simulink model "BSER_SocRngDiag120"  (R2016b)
settings: Solver=FixedStepDiscrete  StartTime=0.0  StopTime=10.0  FixedStep=0.02  RelTol=1e-3  EnableMultiTasking=on
undefined symbols (not defined in the file or in its folder): bin2dec, BSER_cntSocRngDiag_CW, BSER_iSocRngChCurrAccuThres_C, BSER_iSocRngDisCurrAccuThres_C, BSER_rBattSocRngHiFault_C, BSER_rBattSocRngHiWarn_C, BSER_rBattSocRngLoFault_C, BSER_rBattSocRngLoWarn_C, BSER_tiBattSocRngHiFault_C, BSER_tiBattSocRngHiWarn_C, BSER_tiBattSocRngLoFault_C, BSER_tiBattSocRngLoWarn_C, BSPR_iSocRngChrgCurrHi_C, BSPR_iSocRngDisChCurrLo_C, BSPR_tiSocRngCurrCont_C
libraries: simulink x32

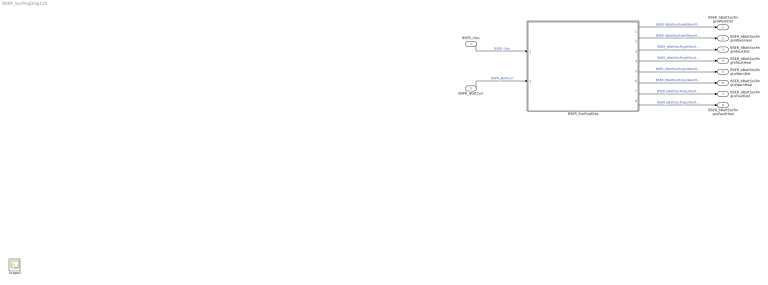
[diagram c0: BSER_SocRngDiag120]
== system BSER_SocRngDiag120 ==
  BSER_rSoc : Inport
  BSPR_iBattCurr : Inport  Port=2
  BSER_SocRngDiag : Subsystem
  BSER_bBattSocRngHiWarnDet : Outport
  BSER_bBattSocRngHiWarnHeal : Outport  Port=2
  BSER_bBattSocRngHiFaultDet : Outport  Port=3
  BSER_bBattSocRngHiFaultHeal : Outport  Port=4
  BSER_bBattSocRngLoWarnDet : Outport  Port=5
  BSER_bBattSocRngLoWarnHeal : Outport  Port=6
  BSER_bBattSocRngLoFaultDet : Outport  Port=7
  BSER_bBattSocRngLoFaultHeal : Outport  Port=8
  Scope2 : Scope
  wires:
  BSER_rSoc/1 -> BSER_SocRngDiag/1(BSER_rSoc)  "BSER_rSoc"
  BSPR_iBattCurr/1 -> BSER_SocRngDiag/2(BSPR_iBattCurr)  "BSPR_iBattCurr"
  BSER_SocRngDiag/1(BSER_bBattSocRngHiWarnDet) -> BSER_bBattSocRngHiWarnDet/1  "BSER_bBattSocRngHiWarnDet"
  BSER_SocRngDiag/2(BSER_bBattSocRngHiWarnHeal) -> BSER_bBattSocRngHiWarnHeal/1  "BSER_bBattSocRngHiWarnHeal"
  BSER_SocRngDiag/3(BSER_bBattSocRngHiFaultDet) -> BSER_bBattSocRngHiFaultDet/1  "BSER_bBattSocRngHiFaultDet"
  BSER_SocRngDiag/4(BSER_bBattSocRngHiFaultHeal) -> BSER_bBattSocRngHiFaultHeal/1  "BSER_bBattSocRngHiFaultHeal"
  BSER_SocRngDiag/5(BSER_bBattSocRngLoWarnDet) -> BSER_bBattSocRngLoWarnDet/1  "BSER_bBattSocRngLoWarnDet"
  BSER_SocRngDiag/6(BSER_bBattSocRngLoWarnHeal) -> BSER_bBattSocRngLoWarnHeal/1  "BSER_bBattSocRngLoWarnHeal"
  BSER_SocRngDiag/7(BSER_bBattSocRngLoFaultDet) -> BSER_bBattSocRngLoFaultDet/1  "BSER_bBattSocRngLoFaultDet"
  BSER_SocRngDiag/8(BSER_bBattSocRngLoFaultHeal) -> BSER_bBattSocRngLoFaultHeal/1  "BSER_bBattSocRngLoFaultHeal"

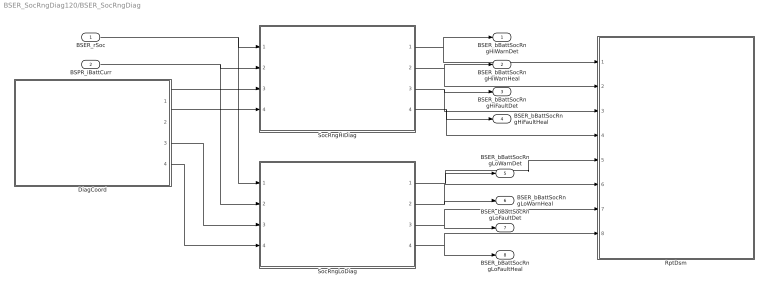
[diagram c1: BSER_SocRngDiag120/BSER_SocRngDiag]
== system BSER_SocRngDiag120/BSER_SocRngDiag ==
  BSER_rSoc : Inport
  BSPR_iBattCurr : Inport  Port=2
  DiagCoord : Subsystem
  RptDsm : Subsystem
  SocRngHiDiag : Subsystem
  SocRngLoDiag : Subsystem
  BSER_bBattSocRngHiWarnDet : Outport
  BSER_bBattSocRngHiWarnHeal : Outport  Port=2
  BSER_bBattSocRngHiFaultDet : Outport  Port=3
  BSER_bBattSocRngHiFaultHeal : Outport  Port=4
  BSER_bBattSocRngLoWarnDet : Outport  Port=5
  BSER_bBattSocRngLoWarnHeal : Outport  Port=6
  BSER_bBattSocRngLoFaultDet : Outport  Port=7
  BSER_bBattSocRngLoFaultHeal : Outport  Port=8
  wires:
  BSER_rSoc/1 -> SocRngHiDiag/1(BSER_rSoc), SocRngLoDiag/1(BSER_rSoc)
  BSPR_iBattCurr/1 -> SocRngHiDiag/2(BSPR_iBattCurr), SocRngLoDiag/2(BSPR_iBattCurr)
  DiagCoord/1(BSPR_bSocRngHiWarnSwt) -> SocRngHiDiag/3(BSPR_bSocRngHiWarnSwt)
  DiagCoord/2(BSPR_bSocRngHiFaultSwt) -> SocRngHiDiag/4(BSPR_bSocRngHiFaultSwt)
  SocRngHiDiag/1(BSER_bBattSocRngHiWarnDet) -> RptDsm/1(BSER_bBattSocRngHiWarnDet), BSER_bBattSocRngHiWarnDet/1
  SocRngHiDiag/2(BSER_bBattSocRngHiWarnHeal) -> RptDsm/2(BSER_bBattSocRngHiWarnHeal), BSER_bBattSocRngHiWarnHeal/1
  DiagCoord/3(BSPR_bSocRngLoWarnSwt) -> SocRngLoDiag/3(BSPR_bSocRngLoWarnSwt)
  DiagCoord/4(BSPR_bSocRngLoFaultSwt) -> SocRngLoDiag/4(BSPR_bSocRngLoFaultSwt)
  SocRngLoDiag/1(BSER_bBattSocRngLoWarnDet) -> RptDsm/5(BSER_bBattSocRngLoWarnDet), BSER_bBattSocRngLoWarnDet/1
  SocRngLoDiag/2(BSER_bBattSocRngLoWarnHeal) -> RptDsm/6(BSER_bBattSocRngLoWarnHeal), BSER_bBattSocRngLoWarnHeal/1
  SocRngHiDiag/3(BSER_bBattSocRngHiFaultDet) -> RptDsm/3(BSER_bBattSocRngHiFaultDet), BSER_bBattSocRngHiFaultDet/1
  SocRngHiDiag/4(BSER_bBattSocRngHiFaultHeal) -> RptDsm/4(BSER_bBattSocRngHiFaultHeal), BSER_bBattSocRngHiFaultHeal/1
  SocRngLoDiag/3(BSER_bBattSocRngLoFaultDet) -> RptDsm/7(BSER_bBattSocRngLoFaultDet), BSER_bBattSocRngLoFaultDet/1
  SocRngLoDiag/4(BSER_bBattSocRngLoFaultHeal) -> BSER_bBattSocRngLoFaultHeal/1, RptDsm/8(BSER_bBattSocRngLoFaultHeal)

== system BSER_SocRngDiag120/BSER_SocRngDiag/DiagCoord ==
  Bitwise Operator : simulink/Logic and Bit Operations/Bitwise Operator  logicop=AND  UseBitMask=on  BitMask=bin2dec('00000001')  BitMaskRealWorld=Stored Integer
  Bitwise Operator1 : simulink/Logic and Bit Operations/Bitwise Operator  logicop=AND  UseBitMask=on  BitMask=bin2dec('00000010')  BitMaskRealWorld=Stored Integer
  Bitwise Operator2 : simulink/Logic and Bit Operations/Bitwise Operator  logicop=AND  UseBitMask=on  BitMask=bin2dec('00000100')  BitMaskRealWorld=Stored Integer
  Bitwise Operator3 : simulink/Logic and Bit Operations/Bitwise Operator  logicop=AND  UseBitMask=on  BitMask=bin2dec('00001000')  BitMaskRealWorld=Stored Integer
  Compare To Constant : simulink/Logic and Bit Operations/Compare To Constant  relop===  const=1  OutDataTypeStr=boolean
  Compare To Constant1 : simulink/Logic and Bit Operations/Compare To Constant  relop===  const=2  OutDataTypeStr=boolean
  Compare To Constant2 : simulink/Logic and Bit Operations/Compare To Constant  relop===  const=4  OutDataTypeStr=boolean
  Compare To Constant3 : simulink/Logic and Bit Operations/Compare To Constant  relop===  const=8  OutDataTypeStr=boolean
  Constant7 : Constant  Value=BSER_cntSocRngDiag_CW
  BSPR_bSocRngHiWarnSwt : Outport
  BSPR_bSocRngHiFaultSwt : Outport  Port=2
  BSPR_bSocRngLoWarnSwt : Outport  Port=3
  BSPR_bSocRngLoFaultSwt : Outport  Port=4
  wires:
  Compare To Constant/1 -> BSPR_bSocRngHiWarnSwt/1  "BSPR_bSocRngHiWarnSwt"
  Compare To Constant1/1 -> BSPR_bSocRngHiFaultSwt/1  "BSPR_bSocRngHiFaultSwt"
  Compare To Constant2/1 -> BSPR_bSocRngLoWarnSwt/1  "BSPR_bSocRngLoWarnSwt"
  Compare To Constant3/1 -> BSPR_bSocRngLoFaultSwt/1  "BSPR_bSocRngLoFaultSwt"
  Constant7/1 -> Bitwise Operator3/1, Bitwise Operator2/1, Bitwise Operator1/1, Bitwise Operator/1
  Bitwise Operator/1 -> Compare To Constant/1
  Bitwise Operator1/1 -> Compare To Constant1/1
  Bitwise Operator2/1 -> Compare To Constant2/1
  Bitwise Operator3/1 -> Compare To Constant3/1

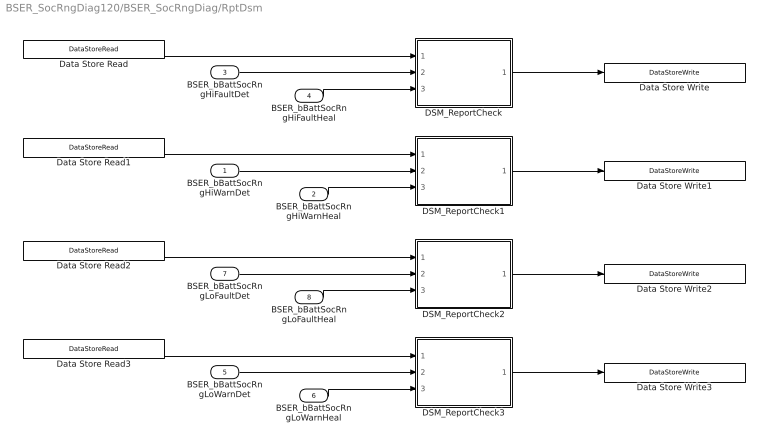
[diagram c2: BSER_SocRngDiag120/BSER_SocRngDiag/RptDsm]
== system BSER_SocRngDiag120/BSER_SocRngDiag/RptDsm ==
  BSER_bBattSocRngHiWarnDet : Inport
  BSER_bBattSocRngHiWarnHeal : Inport  Port=2
  BSER_bBattSocRngHiFaultDet : Inport  Port=3
  BSER_bBattSocRngHiFaultHeal : Inport  Port=4
  BSER_bBattSocRngLoWarnDet : Inport  Port=5
  BSER_bBattSocRngLoWarnHeal : Inport  Port=6
  BSER_bBattSocRngLoFaultDet : Inport  Port=7
  BSER_bBattSocRngLoFaultHeal : Inport  Port=8
  DSM_ReportCheck : Subsystem  TreatAsAtomicUnit=on  RTWFcnName=DSM_ReportCheck  RTWFileName=SrvLib
  DSM_ReportCheck1 : Subsystem  TreatAsAtomicUnit=on  RTWFcnName=DSM_ReportCheck  RTWFileName=SrvLib
  DSM_ReportCheck2 : Subsystem  TreatAsAtomicUnit=on  RTWFcnName=DSM_ReportCheck  RTWFileName=SrvLib
  DSM_ReportCheck3 : Subsystem  TreatAsAtomicUnit=on  RTWFcnName=DSM_ReportCheck  RTWFileName=SrvLib
  Data Store Read : DataStoreRead  DataStoreName=DFC_SocRngHiMax
  Data Store Read1 : DataStoreRead  DataStoreName=DFC_SocRngHiMin
  Data Store Read2 : DataStoreRead  DataStoreName=DFC_SocRngLoMax
  Data Store Read3 : DataStoreRead  DataStoreName=DFC_SocRngLoMin
  Data Store Write : DataStoreWrite  DataStoreName=DFC_SocRngHiMax
  Data Store Write1 : DataStoreWrite  DataStoreName=DFC_SocRngHiMin
  Data Store Write2 : DataStoreWrite  DataStoreName=DFC_SocRngLoMax
  Data Store Write3 : DataStoreWrite  DataStoreName=DFC_SocRngLoMin
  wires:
  BSER_bBattSocRngHiFaultHeal/1 -> DSM_ReportCheck/3(Heal)
  BSER_bBattSocRngHiFaultDet/1 -> DSM_ReportCheck/2(Err)
  BSER_bBattSocRngHiWarnHeal/1 -> DSM_ReportCheck1/3(Heal)
  BSER_bBattSocRngHiWarnDet/1 -> DSM_ReportCheck1/2(Err)
  BSER_bBattSocRngLoWarnDet/1 -> DSM_ReportCheck3/2(Err)
  BSER_bBattSocRngLoWarnHeal/1 -> DSM_ReportCheck3/3(Heal)
  BSER_bBattSocRngLoFaultDet/1 -> DSM_ReportCheck2/2(Err)
  BSER_bBattSocRngLoFaultHeal/1 -> DSM_ReportCheck2/3(Heal)
  Data Store Read/1 -> DSM_ReportCheck/1(Dfc_id_nv)
  Data Store Read1/1 -> DSM_ReportCheck1/1(Dfc_id_nv)
  Data Store Read2/1 -> DSM_ReportCheck2/1(Dfc_id_nv)
  Data Store Read3/1 -> DSM_ReportCheck3/1(Dfc_id_nv)
  DSM_ReportCheck/1(Dfc_id) -> Data Store Write/1
  DSM_ReportCheck1/1(Dfc_id) -> Data Store Write1/1
  DSM_ReportCheck2/1(Dfc_id) -> Data Store Write2/1
  DSM_ReportCheck3/1(Dfc_id) -> Data Store Write3/1

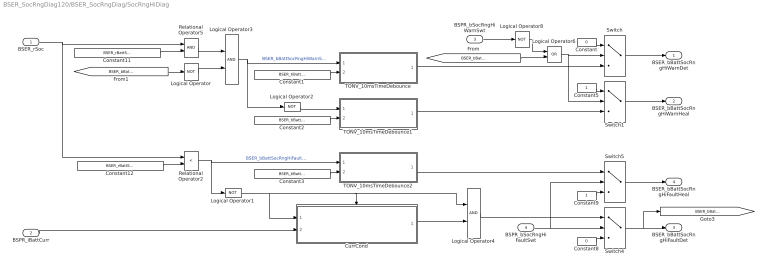
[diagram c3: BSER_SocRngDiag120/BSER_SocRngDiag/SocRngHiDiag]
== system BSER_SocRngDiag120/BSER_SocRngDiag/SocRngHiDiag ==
  BSER_rSoc : Inport
  BSPR_iBattCurr : Inport  Port=2
  BSPR_bSocRngHiWarnSwt : Inport  Port=3
  BSPR_bSocRngHiFaultSwt : Inport  Port=4
  Constant : Constant  Value=0  OutDataTypeStr=boolean
  Constant1 : Constant  Value=BSER_tiBattSocRngHiWarn_C
  Constant11 : Constant  Value=BSER_rBattSocRngHiWarn_C
  Constant12 : Constant  Value=BSER_rBattSocRngHiFault_C
  Constant2 : Constant  Value=BSER_tiBattSocRngHiWarn_C
  Constant3 : Constant  Value=BSER_tiBattSocRngHiFault_C
  Constant5 : Constant  OutDataTypeStr=boolean
  Constant8 : Constant  Value=0  OutDataTypeStr=boolean
  Constant9 : Constant  OutDataTypeStr=boolean
  CurrCond : Subsystem
  Logical Operator{,1..2,8} (4 alike) : Logic  Operator=NOT  AllPortsSameDT=off  OutDataTypeStr=boolean
  Logical Operator3 : Logic  AllPortsSameDT=off  OutDataTypeStr=boolean
  Logical Operator4 : Logic  AllPortsSameDT=off  OutDataTypeStr=boolean
  Logical Operator6 : Logic  Operator=OR  AllPortsSameDT=off  OutDataTypeStr=boolean
  Relational Operator2 : RelationalOperator  Operator=<  OutDataTypeStr=boolean  RndMeth=Simplest
  Relational Operator5 : RelationalOperator  OutDataTypeStr=boolean  RndMeth=Simplest
  Switch{,1,4..5} (4 alike) : Switch  Criteria=u2 > Threshold
  TONV_10msTimeDebounce : Subsystem  TreatAsAtomicUnit=on  RTWFcnName=TONV_10msTimeDebounce  RTWFileName=SrvLib
  TONV_10msTimeDebounce1 : Subsystem  TreatAsAtomicUnit=on  RTWFcnName=TONV_10msTimeDebounce  RTWFileName=SrvLib
  TONV_10msTimeDebounce2 : Subsystem  TreatAsAtomicUnit=on  RTWFcnName=TONV_10msTimeDebounce  RTWFileName=SrvLib
  BSER_bBattSocRngHiWarnDet : Outport
  BSER_bBattSocRngHiWarnHeal : Outport  Port=2
  BSER_bBattSocRngHiFaultDet : Outport  Port=3
  BSER_bBattSocRngHiFaultHeal : Outport  Port=4
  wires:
  BSER_rSoc/1 -> Relational Operator2/1, Relational Operator5/1
  Constant11/1 -> Relational Operator5/2
  Constant1/1 -> TONV_10msTimeDebounce/2(T)
  Constant12/1 -> Relational Operator2/2
  Relational Operator5/1 -> Logical Operator3/1
  Logical Operator3/1 -> TONV_10msTimeDebounce/1(u), Logical Operator2/1  "BSER_bBattSocRngHiWarnStt"
  Constant2/1 -> TONV_10msTimeDebounce1/2(T)
  Logical Operator2/1 -> TONV_10msTimeDebounce1/1(u)
  Switch/1 -> BSER_bBattSocRngHiWarnDet/1
  Switch1/1 -> BSER_bBattSocRngHiWarnHeal/1
  TONV_10msTimeDebounce1/1(y) -> Switch1/3
  Logical Operator4/1 -> Switch4/1
  Constant8/1 -> Switch4/3
  TONV_10msTimeDebounce2/1(y) -> Switch5/1
  Constant9/1 -> Switch5/3
  Switch5/1 -> BSER_bBattSocRngHiFaultHeal/1
  Switch4/1 -> [BSER_bBattSocRngHiFaultDet], BSER_bBattSocRngHiFaultDet/1
  Logical Operator6/1 -> Switch1/2, Switch/2
  [BSER_bBattSocRngHiFaultDet] -> Logical Operator6/2
  Logical Operator8/1 -> Logical Operator6/1
  Constant/1 -> Switch/1
  TONV_10msTimeDebounce/1(y) -> Switch/3
  Constant5/1 -> Switch1/1
  Logical Operator/1 -> Logical Operator3/2
  BSPR_bSocRngHiWarnSwt/1 -> Logical Operator8/1
  [BSER_bBattSocRngHiFaultDet] -> Logical Operator/1
  BSPR_bSocRngHiFaultSwt/1 -> Switch5/2, Switch4/2
  Relational Operator2/1 -> TONV_10msTimeDebounce2/1(u), Logical Operator1/1  "BSER_bBattSocRngHiFaultStt"
  Constant3/1 -> TONV_10msTimeDebounce2/2(T)
  BSPR_iBattCurr/1 -> CurrCond/2(BSPR_iBattCurr)
  CurrCond/1(BSPR_bSocRngChrgCurrCond) -> Logical Operator4/2
  Logical Operator1/1 -> CurrCond/1(BSER_bBattSocRngHiFaultStt), CurrCond/Enable, Logical Operator4/1

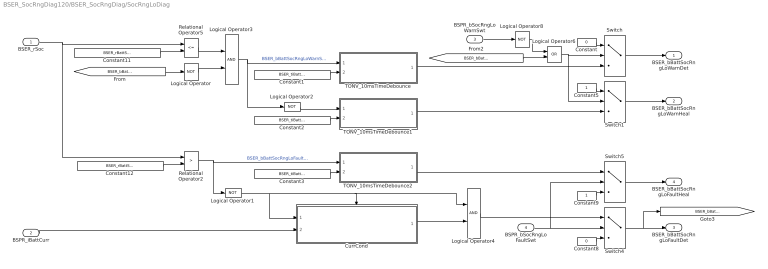
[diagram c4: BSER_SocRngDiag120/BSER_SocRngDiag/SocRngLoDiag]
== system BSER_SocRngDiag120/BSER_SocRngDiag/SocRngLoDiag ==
  BSER_rSoc : Inport
  BSPR_iBattCurr : Inport  Port=2
  BSPR_bSocRngLoWarnSwt : Inport  Port=3
  BSPR_bSocRngLoFaultSwt : Inport  Port=4
  Constant : Constant  Value=0  OutDataTypeStr=boolean
  Constant1 : Constant  Value=BSER_tiBattSocRngLoWarn_C
  Constant11 : Constant  Value=BSER_rBattSocRngLoWarn_C
  Constant12 : Constant  Value=BSER_rBattSocRngLoFault_C
  Constant2 : Constant  Value=BSER_tiBattSocRngLoWarn_C
  Constant3 : Constant  Value=BSER_tiBattSocRngLoFault_C
  Constant5 : Constant  OutDataTypeStr=boolean
  Constant8 : Constant  Value=0  OutDataTypeStr=boolean
  Constant9 : Constant  OutDataTypeStr=boolean
  CurrCond : Subsystem
  Logical Operator{,1..2,8} (4 alike) : Logic  Operator=NOT  AllPortsSameDT=off  OutDataTypeStr=boolean
  Logical Operator3 : Logic  AllPortsSameDT=off  OutDataTypeStr=boolean
  Logical Operator4 : Logic  AllPortsSameDT=off  OutDataTypeStr=boolean
  Logical Operator6 : Logic  Operator=OR  AllPortsSameDT=off  OutDataTypeStr=boolean
  Relational Operator2 : RelationalOperator  Operator=>  OutDataTypeStr=boolean  RndMeth=Simplest
  Relational Operator5 : RelationalOperator  Operator=<=  OutDataTypeStr=boolean  RndMeth=Simplest
  Switch{,1,4..5} (4 alike) : Switch  Criteria=u2 > Threshold
  TONV_10msTimeDebounce : Subsystem  TreatAsAtomicUnit=on  RTWFcnName=TONV_10msTimeDebounce  RTWFileName=SrvLib
  TONV_10msTimeDebounce1 : Subsystem  TreatAsAtomicUnit=on  RTWFcnName=TONV_10msTimeDebounce  RTWFileName=SrvLib
  TONV_10msTimeDebounce2 : Subsystem  TreatAsAtomicUnit=on  RTWFcnName=TONV_10msTimeDebounce  RTWFileName=SrvLib
  BSER_bBattSocRngLoWarnDet : Outport
  BSER_bBattSocRngLoWarnHeal : Outport  Port=2
  BSER_bBattSocRngLoFaultDet : Outport  Port=3
  BSER_bBattSocRngLoFaultHeal : Outport  Port=4
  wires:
  Logical Operator1/1 -> CurrCond/1(BSER_bBattSocRngLo), CurrCond/Enable, Logical Operator4/1
  CurrCond/1(BSPR_bSocRngDisChCurrCond) -> Logical Operator4/2
  BSPR_iBattCurr/1 -> CurrCond/2(BSPR_iBattCurr)
  Constant3/1 -> TONV_10msTimeDebounce2/2(T)
  Relational Operator2/1 -> TONV_10msTimeDebounce2/1(u), Logical Operator1/1  "BSER_bBattSocRngLoFaultStt"
  BSPR_bSocRngLoFaultSwt/1 -> Switch4/2, Switch5/2
  [BSER_bBattSocRngLoFaultDet] -> Logical Operator/1
  BSPR_bSocRngLoWarnSwt/1 -> Logical Operator8/1
  Logical Operator/1 -> Logical Operator3/2
  Constant5/1 -> Switch1/1
  TONV_10msTimeDebounce/1(y) -> Switch/3
  Constant/1 -> Switch/1
  Logical Operator8/1 -> Logical Operator6/1
  [BSER_bBattSocRngLoFaultDet] -> Logical Operator6/2
  Logical Operator6/1 -> Switch/2, Switch1/2
  Switch4/1 -> BSER_bBattSocRngLoFaultDet/1, [BSER_bBattSocRngLoFaultDet]
  Switch5/1 -> BSER_bBattSocRngLoFaultHeal/1
  Constant9/1 -> Switch5/3
  TONV_10msTimeDebounce2/1(y) -> Switch5/1
  Constant8/1 -> Switch4/3
  Logical Operator4/1 -> Switch4/1
  TONV_10msTimeDebounce1/1(y) -> Switch1/3
  Switch1/1 -> BSER_bBattSocRngLoWarnHeal/1
  Switch/1 -> BSER_bBattSocRngLoWarnDet/1
  Logical Operator2/1 -> TONV_10msTimeDebounce1/1(u)
  Constant2/1 -> TONV_10msTimeDebounce1/2(T)
  Logical Operator3/1 -> TONV_10msTimeDebounce/1(u), Logical Operator2/1  "BSER_bBattSocRngLoWarnStt"
  Relational Operator5/1 -> Logical Operator3/1
  Constant12/1 -> Relational Operator2/2
  Constant1/1 -> TONV_10msTimeDebounce/2(T)
  Constant11/1 -> Relational Operator5/2
  BSER_rSoc/1 -> Relational Operator5/1, Relational Operator2/1

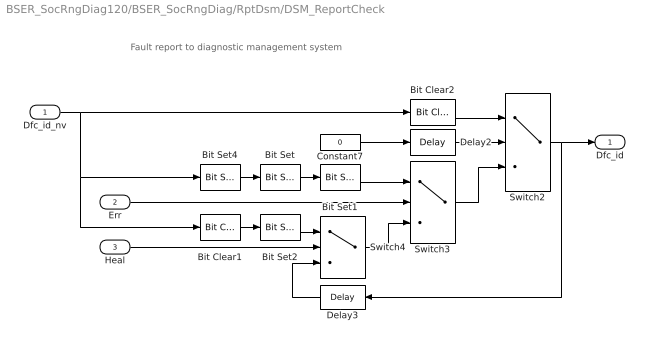
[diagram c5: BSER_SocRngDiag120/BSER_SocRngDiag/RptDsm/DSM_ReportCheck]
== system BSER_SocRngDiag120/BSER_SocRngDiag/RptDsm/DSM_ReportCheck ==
  note: Fault report to diagnostic management system
  Dfc_id_nv : Inport  OutDataTypeStr=uint8
  Err : Inport  Port=2
  Heal : Inport  Port=3
  Bit Clear1 : simulink/Logic and Bit Operations/Bit Clear  iBit=4
  Bit Clear2 : simulink/Logic and Bit Operations/Bit Clear  iBit=3
  Bit Set : simulink/Logic and Bit Operations/Bit Set  iBit=4
  Bit Set1 : simulink/Logic and Bit Operations/Bit Set  iBit=3
  Bit Set2 : simulink/Logic and Bit Operations/Bit Set  iBit=3
  Bit Set4 : simulink/Logic and Bit Operations/Bit Set  iBit=7
  Constant7 : Constant  Value=0  OutDataTypeStr=boolean
  Delay2 : Delay  DelayLength=1  InitialCondition=1
  Delay3 : Delay  DelayLength=1  InitialCondition=0
  Switch2 : Switch  Criteria=u2 ~= 0
  Switch3 : Switch  Criteria=u2 ~= 0
  Switch4 : Switch  Criteria=u2 ~= 0
  Dfc_id : Outport  OutDataTypeStr=uint8
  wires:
  Dfc_id_nv/1 -> Bit Clear2/1, Bit Set4/1, Bit Clear1/1
  Bit Set4/1 -> Bit Set/1
  Constant7/1 -> Delay2/1
  Delay2/1 -> Switch2/2
  Switch3/1 -> Switch2/3
  Bit Clear2/1 -> Switch2/1
  Switch2/1 -> Delay3/1, Dfc_id/1
  Bit Set1/1 -> Switch3/1
  Bit Set/1 -> Bit Set1/1
  Switch4/1 -> Switch3/3
  Err/1 -> Switch3/2
  Bit Set2/1 -> Switch4/1
  Bit Clear1/1 -> Bit Set2/1
  Delay3/1 -> Switch4/3
  Heal/1 -> Switch4/2

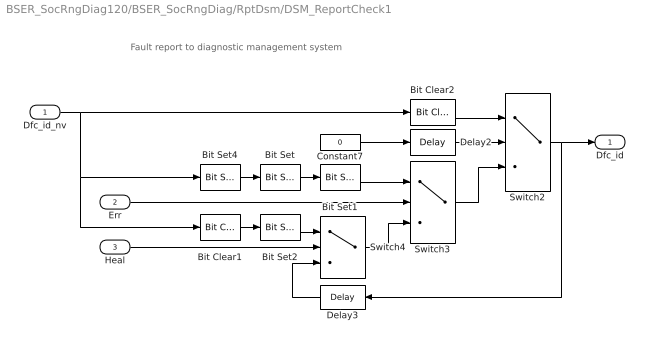
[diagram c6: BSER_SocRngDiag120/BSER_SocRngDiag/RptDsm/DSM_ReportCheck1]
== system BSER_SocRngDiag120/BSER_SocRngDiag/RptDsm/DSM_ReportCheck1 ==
  note: Fault report to diagnostic management system
  Dfc_id_nv : Inport  OutDataTypeStr=uint8
  Err : Inport  Port=2
  Heal : Inport  Port=3
  Bit Clear1 : simulink/Logic and Bit Operations/Bit Clear  iBit=4
  Bit Clear2 : simulink/Logic and Bit Operations/Bit Clear  iBit=3
  Bit Set : simulink/Logic and Bit Operations/Bit Set  iBit=4
  Bit Set1 : simulink/Logic and Bit Operations/Bit Set  iBit=3
  Bit Set2 : simulink/Logic and Bit Operations/Bit Set  iBit=3
  Bit Set4 : simulink/Logic and Bit Operations/Bit Set  iBit=7
  Constant7 : Constant  Value=0  OutDataTypeStr=boolean
  Delay2 : Delay  DelayLength=1  InitialCondition=1
  Delay3 : Delay  DelayLength=1  InitialCondition=0
  Switch2 : Switch  Criteria=u2 ~= 0
  Switch3 : Switch  Criteria=u2 ~= 0
  Switch4 : Switch  Criteria=u2 ~= 0
  Dfc_id : Outport  OutDataTypeStr=uint8
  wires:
  Heal/1 -> Switch4/2
  Delay3/1 -> Switch4/3
  Bit Clear1/1 -> Bit Set2/1
  Bit Set2/1 -> Switch4/1
  Err/1 -> Switch3/2
  Switch4/1 -> Switch3/3
  Bit Set/1 -> Bit Set1/1
  Bit Set1/1 -> Switch3/1
  Switch2/1 -> Dfc_id/1, Delay3/1
  Bit Clear2/1 -> Switch2/1
  Switch3/1 -> Switch2/3
  Delay2/1 -> Switch2/2
  Constant7/1 -> Delay2/1
  Bit Set4/1 -> Bit Set/1
  Dfc_id_nv/1 -> Bit Clear1/1, Bit Set4/1, Bit Clear2/1

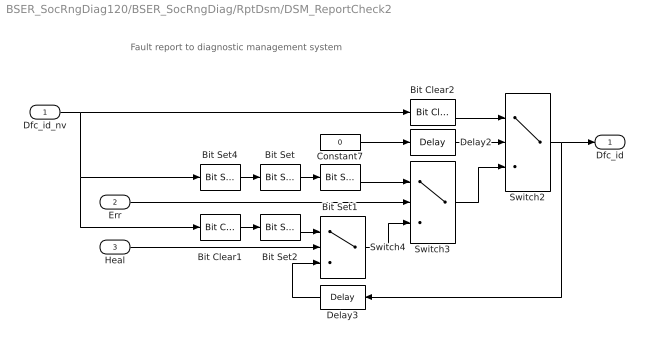
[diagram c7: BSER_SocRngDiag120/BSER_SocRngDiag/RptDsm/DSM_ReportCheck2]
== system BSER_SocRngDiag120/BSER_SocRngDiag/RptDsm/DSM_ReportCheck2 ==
  note: Fault report to diagnostic management system
  Dfc_id_nv : Inport  OutDataTypeStr=uint8
  Err : Inport  Port=2
  Heal : Inport  Port=3
  Bit Clear1 : simulink/Logic and Bit Operations/Bit Clear  iBit=4
  Bit Clear2 : simulink/Logic and Bit Operations/Bit Clear  iBit=3
  Bit Set : simulink/Logic and Bit Operations/Bit Set  iBit=4
  Bit Set1 : simulink/Logic and Bit Operations/Bit Set  iBit=3
  Bit Set2 : simulink/Logic and Bit Operations/Bit Set  iBit=3
  Bit Set4 : simulink/Logic and Bit Operations/Bit Set  iBit=7
  Constant7 : Constant  Value=0  OutDataTypeStr=boolean
  Delay2 : Delay  DelayLength=1  InitialCondition=1
  Delay3 : Delay  DelayLength=1  InitialCondition=0
  Switch2 : Switch  Criteria=u2 ~= 0
  Switch3 : Switch  Criteria=u2 ~= 0
  Switch4 : Switch  Criteria=u2 ~= 0
  Dfc_id : Outport  OutDataTypeStr=uint8
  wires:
  Dfc_id_nv/1 -> Bit Clear2/1, Bit Set4/1, Bit Clear1/1
  Bit Set4/1 -> Bit Set/1
  Constant7/1 -> Delay2/1
  Delay2/1 -> Switch2/2
  Switch3/1 -> Switch2/3
  Bit Clear2/1 -> Switch2/1
  Switch2/1 -> Delay3/1, Dfc_id/1
  Bit Set1/1 -> Switch3/1
  Bit Set/1 -> Bit Set1/1
  Switch4/1 -> Switch3/3
  Err/1 -> Switch3/2
  Bit Set2/1 -> Switch4/1
  Bit Clear1/1 -> Bit Set2/1
  Delay3/1 -> Switch4/3
  Heal/1 -> Switch4/2

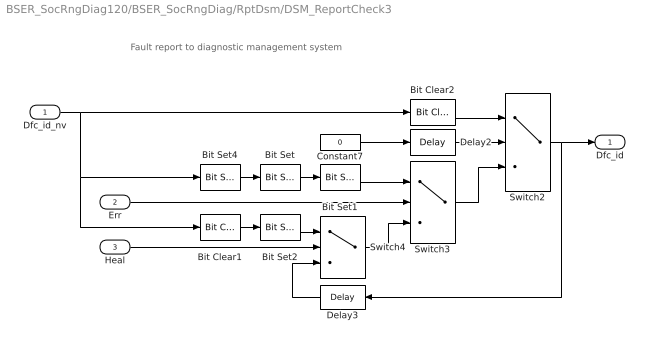
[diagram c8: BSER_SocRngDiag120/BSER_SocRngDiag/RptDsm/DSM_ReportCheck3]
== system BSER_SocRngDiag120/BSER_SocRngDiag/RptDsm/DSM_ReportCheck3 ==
  note: Fault report to diagnostic management system
  Dfc_id_nv : Inport  OutDataTypeStr=uint8
  Err : Inport  Port=2
  Heal : Inport  Port=3
  Bit Clear1 : simulink/Logic and Bit Operations/Bit Clear  iBit=4
  Bit Clear2 : simulink/Logic and Bit Operations/Bit Clear  iBit=3
  Bit Set : simulink/Logic and Bit Operations/Bit Set  iBit=4
  Bit Set1 : simulink/Logic and Bit Operations/Bit Set  iBit=3
  Bit Set2 : simulink/Logic and Bit Operations/Bit Set  iBit=3
  Bit Set4 : simulink/Logic and Bit Operations/Bit Set  iBit=7
  Constant7 : Constant  Value=0  OutDataTypeStr=boolean
  Delay2 : Delay  DelayLength=1  InitialCondition=1
  Delay3 : Delay  DelayLength=1  InitialCondition=0
  Switch2 : Switch  Criteria=u2 ~= 0
  Switch3 : Switch  Criteria=u2 ~= 0
  Switch4 : Switch  Criteria=u2 ~= 0
  Dfc_id : Outport  OutDataTypeStr=uint8
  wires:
  Heal/1 -> Switch4/2
  Delay3/1 -> Switch4/3
  Bit Clear1/1 -> Bit Set2/1
  Bit Set2/1 -> Switch4/1
  Err/1 -> Switch3/2
  Switch4/1 -> Switch3/3
  Bit Set/1 -> Bit Set1/1
  Bit Set1/1 -> Switch3/1
  Switch2/1 -> Dfc_id/1, Delay3/1
  Bit Clear2/1 -> Switch2/1
  Switch3/1 -> Switch2/3
  Delay2/1 -> Switch2/2
  Constant7/1 -> Delay2/1
  Bit Set4/1 -> Bit Set/1
  Dfc_id_nv/1 -> Bit Clear1/1, Bit Set4/1, Bit Clear2/1

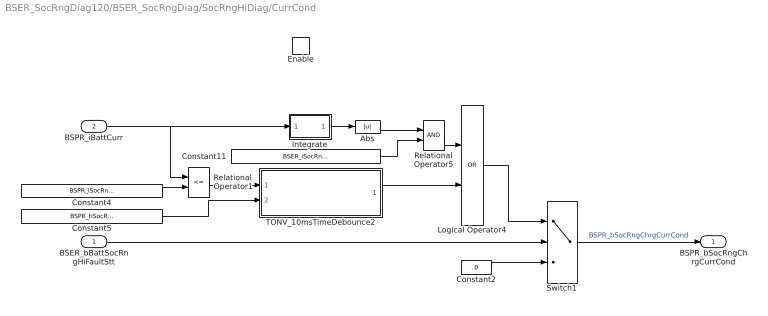
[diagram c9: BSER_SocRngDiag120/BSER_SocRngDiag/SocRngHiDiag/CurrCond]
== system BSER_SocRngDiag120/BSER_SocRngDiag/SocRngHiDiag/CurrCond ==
  BSER_bBattSocRngHiFaultStt : Inport
  BSPR_iBattCurr : Inport  Port=2
  Enable : EnablePort  StatesWhenEnabling=reset
  Abs : Abs
  Constant11 : Constant  Value=BSER_iSocRngChCurrAccuThres_C
  Constant2 : Constant  Value=0  OutDataTypeStr=boolean
  Constant4 : Constant  Value=BSPR_iSocRngChrgCurrHi_C
  Constant5 : Constant  Value=BSPR_tiSocRngCurrCont_C
  Integrate : Subsystem
  Logical Operator4 : Logic  Operator=OR  AllPortsSameDT=off  OutDataTypeStr=boolean
  Relational Operator1 : RelationalOperator  Operator=<=  OutDataTypeStr=boolean  RndMeth=Simplest
  Relational Operator5 : RelationalOperator  OutDataTypeStr=boolean  RndMeth=Simplest
  Switch1 : Switch  Criteria=u2 > Threshold
  TONV_10msTimeDebounce2 : Subsystem  TreatAsAtomicUnit=on  RTWFcnName=TONV_10msTimeDebounce  RTWFileName=SrvLib
  BSPR_bSocRngChrgCurrCond : Outport  InitialOutput=[0]
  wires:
  Integrate/1(Out) -> Abs/1
  Constant11/1 -> Relational Operator5/2
  Constant5/1 -> TONV_10msTimeDebounce2/2(T)
  Constant4/1 -> Relational Operator1/2
  Relational Operator1/1 -> TONV_10msTimeDebounce2/1(u)
  BSER_bBattSocRngHiFaultStt/1 -> Switch1/2
  Constant2/1 -> Switch1/3
  Switch1/1 -> BSPR_bSocRngChrgCurrCond/1  "BSPR_bSocRngChrgCurrCond"
  Logical Operator4/1 -> Switch1/1
  TONV_10msTimeDebounce2/1(y) -> Logical Operator4/2
  Relational Operator5/1 -> Logical Operator4/1
  BSPR_iBattCurr/1 -> Integrate/1(In), Relational Operator1/1
  Abs/1 -> Relational Operator5/1

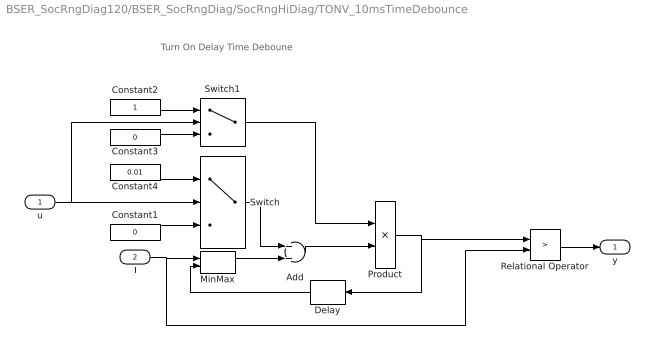
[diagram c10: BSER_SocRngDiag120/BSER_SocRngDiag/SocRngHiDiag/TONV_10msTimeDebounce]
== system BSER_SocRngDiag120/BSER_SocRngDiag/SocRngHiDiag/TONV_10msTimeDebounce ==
  note: Turn On Delay Time Deboune
  u : Inport
  T : Inport  Port=2
  Add : Sum
  Constant1 : Constant  Value=0  OutDataTypeStr=single
  Constant2 : Constant  OutDataTypeStr=uint8
  Constant3 : Constant  Value=0  OutDataTypeStr=uint8
  Constant4 : Constant  Value=0.01  OutDataTypeStr=single
  Delay : Delay  DelayLength=1  InitialCondition=0
  MinMax : MinMax  Inputs=2
  Product : Product  OutMin=[0]  OutMax=[65535]  OutDataTypeStr=single
  Relational Operator : RelationalOperator  Operator=>  OutDataTypeStr=boolean  RndMeth=Simplest
  Switch : Switch  Criteria=u2 ~= 0
  Switch1 : Switch  Criteria=u2 ~= 0
  y : Outport
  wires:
  MinMax/1 -> Add/2
  T/1 -> Relational Operator/2, MinMax/1
  Relational Operator/1 -> y/1
  Delay/1 -> MinMax/2
  Switch/1 -> Add/1
  Product/1 -> Delay/1, Relational Operator/1
  Add/1 -> Product/2
  Constant1/1 -> Switch/3
  Constant4/1 -> Switch/1
  u/1 -> Switch/2, Switch1/2
  Constant2/1 -> Switch1/1
  Constant3/1 -> Switch1/3
  Switch1/1 -> Product/1

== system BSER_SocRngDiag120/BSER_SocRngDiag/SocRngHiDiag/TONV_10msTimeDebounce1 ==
  note: Turn On Delay Time Deboune
  u : Inport
  T : Inport  Port=2
  Add : Sum
  Constant1 : Constant  Value=0  OutDataTypeStr=single
  Constant2 : Constant  OutDataTypeStr=uint8
  Constant3 : Constant  Value=0  OutDataTypeStr=uint8
  Constant4 : Constant  Value=0.01  OutDataTypeStr=single
  Delay : Delay  DelayLength=1  InitialCondition=0
  MinMax : MinMax  Inputs=2
  Product : Product  OutMin=[0]  OutMax=[65535]  OutDataTypeStr=single
  Relational Operator : RelationalOperator  Operator=>  OutDataTypeStr=boolean  RndMeth=Simplest
  Switch : Switch  Criteria=u2 ~= 0
  Switch1 : Switch  Criteria=u2 ~= 0
  y : Outport
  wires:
  Switch1/1 -> Product/1
  Constant3/1 -> Switch1/3
  Constant2/1 -> Switch1/1
  u/1 -> Switch1/2, Switch/2
  Constant4/1 -> Switch/1
  Constant1/1 -> Switch/3
  Add/1 -> Product/2
  Product/1 -> Relational Operator/1, Delay/1
  Switch/1 -> Add/1
  Delay/1 -> MinMax/2
  Relational Operator/1 -> y/1
  T/1 -> MinMax/1, Relational Operator/2
  MinMax/1 -> Add/2

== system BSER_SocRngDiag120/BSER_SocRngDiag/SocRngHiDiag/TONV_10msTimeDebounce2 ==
  note: Turn On Delay Time Deboune
  u : Inport
  T : Inport  Port=2
  Add : Sum
  Constant1 : Constant  Value=0  OutDataTypeStr=single
  Constant2 : Constant  OutDataTypeStr=uint8
  Constant3 : Constant  Value=0  OutDataTypeStr=uint8
  Constant4 : Constant  Value=0.01  OutDataTypeStr=single
  Delay : Delay  DelayLength=1  InitialCondition=0
  MinMax : MinMax  Inputs=2
  Product : Product  OutMin=[0]  OutMax=[65535]  OutDataTypeStr=single
  Relational Operator : RelationalOperator  Operator=>  OutDataTypeStr=boolean  RndMeth=Simplest
  Switch : Switch  Criteria=u2 ~= 0
  Switch1 : Switch  Criteria=u2 ~= 0
  y : Outport
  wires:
  MinMax/1 -> Add/2
  T/1 -> Relational Operator/2, MinMax/1
  Relational Operator/1 -> y/1
  Delay/1 -> MinMax/2
  Switch/1 -> Add/1
  Product/1 -> Delay/1, Relational Operator/1
  Add/1 -> Product/2
  Constant1/1 -> Switch/3
  Constant4/1 -> Switch/1
  u/1 -> Switch/2, Switch1/2
  Constant2/1 -> Switch1/1
  Constant3/1 -> Switch1/3
  Switch1/1 -> Product/1

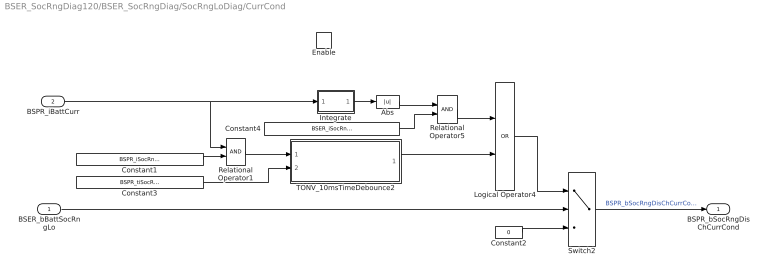
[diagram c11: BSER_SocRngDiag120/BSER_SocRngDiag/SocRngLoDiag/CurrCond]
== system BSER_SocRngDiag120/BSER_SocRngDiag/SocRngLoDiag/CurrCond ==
  BSER_bBattSocRngLo : Inport
  BSPR_iBattCurr : Inport  Port=2
  Enable : EnablePort  StatesWhenEnabling=reset
  Abs : Abs
  Constant1 : Constant  Value=BSPR_iSocRngDisChCurrLo_C
  Constant2 : Constant  Value=0  OutDataTypeStr=boolean
  Constant3 : Constant  Value=BSPR_tiSocRngCurrCont_C
  Constant4 : Constant  Value=BSER_iSocRngDisCurrAccuThres_C
  Integrate : Subsystem
  Logical Operator4 : Logic  Operator=OR  AllPortsSameDT=off  OutDataTypeStr=boolean
  Relational Operator1 : RelationalOperator  OutDataTypeStr=boolean  RndMeth=Simplest
  Relational Operator5 : RelationalOperator  OutDataTypeStr=boolean  RndMeth=Simplest
  Switch2 : Switch  Criteria=u2 > Threshold
  TONV_10msTimeDebounce2 : Subsystem  TreatAsAtomicUnit=on  RTWFcnName=TONV_10msTimeDebounce  RTWFileName=SrvLib
  BSPR_bSocRngDisChCurrCond : Outport  InitialOutput=[0]
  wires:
  Relational Operator5/1 -> Logical Operator4/1
  TONV_10msTimeDebounce2/1(y) -> Logical Operator4/2
  Logical Operator4/1 -> Switch2/1
  Switch2/1 -> BSPR_bSocRngDisChCurrCond/1  "BSPR_bSocRngDisChCurrCond"
  Constant2/1 -> Switch2/3
  BSER_bBattSocRngLo/1 -> Switch2/2
  Relational Operator1/1 -> TONV_10msTimeDebounce2/1(u)
  Constant1/1 -> Relational Operator1/2
  Constant3/1 -> TONV_10msTimeDebounce2/2(T)
  Constant4/1 -> Relational Operator5/2
  Integrate/1(Out) -> Abs/1
  BSPR_iBattCurr/1 -> Integrate/1(In), Relational Operator1/1
  Abs/1 -> Relational Operator5/1

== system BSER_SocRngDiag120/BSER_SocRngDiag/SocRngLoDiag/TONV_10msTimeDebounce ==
  note: Turn On Delay Time Deboune
  u : Inport
  T : Inport  Port=2
  Add : Sum
  Constant1 : Constant  Value=0  OutDataTypeStr=single
  Constant2 : Constant  OutDataTypeStr=uint8
  Constant3 : Constant  Value=0  OutDataTypeStr=uint8
  Constant4 : Constant  Value=0.01  OutDataTypeStr=single
  Delay : Delay  DelayLength=1  InitialCondition=0
  MinMax : MinMax  Inputs=2
  Product : Product  OutMin=[0]  OutMax=[65535]  OutDataTypeStr=single
  Relational Operator : RelationalOperator  Operator=>  OutDataTypeStr=boolean  RndMeth=Simplest
  Switch : Switch  Criteria=u2 ~= 0
  Switch1 : Switch  Criteria=u2 ~= 0
  y : Outport
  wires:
  MinMax/1 -> Add/2
  T/1 -> Relational Operator/2, MinMax/1
  Relational Operator/1 -> y/1
  Delay/1 -> MinMax/2
  Switch/1 -> Add/1
  Product/1 -> Delay/1, Relational Operator/1
  Add/1 -> Product/2
  Constant1/1 -> Switch/3
  Constant4/1 -> Switch/1
  u/1 -> Switch/2, Switch1/2
  Constant2/1 -> Switch1/1
  Constant3/1 -> Switch1/3
  Switch1/1 -> Product/1

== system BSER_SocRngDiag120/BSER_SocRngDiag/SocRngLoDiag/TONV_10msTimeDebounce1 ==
  note: Turn On Delay Time Deboune
  u : Inport
  T : Inport  Port=2
  Add : Sum
  Constant1 : Constant  Value=0  OutDataTypeStr=single
  Constant2 : Constant  OutDataTypeStr=uint8
  Constant3 : Constant  Value=0  OutDataTypeStr=uint8
  Constant4 : Constant  Value=0.01  OutDataTypeStr=single
  Delay : Delay  DelayLength=1  InitialCondition=0
  MinMax : MinMax  Inputs=2
  Product : Product  OutMin=[0]  OutMax=[65535]  OutDataTypeStr=single
  Relational Operator : RelationalOperator  Operator=>  OutDataTypeStr=boolean  RndMeth=Simplest
  Switch : Switch  Criteria=u2 ~= 0
  Switch1 : Switch  Criteria=u2 ~= 0
  y : Outport
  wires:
  Switch1/1 -> Product/1
  Constant3/1 -> Switch1/3
  Constant2/1 -> Switch1/1
  u/1 -> Switch1/2, Switch/2
  Constant4/1 -> Switch/1
  Constant1/1 -> Switch/3
  Add/1 -> Product/2
  Product/1 -> Relational Operator/1, Delay/1
  Switch/1 -> Add/1
  Delay/1 -> MinMax/2
  Relational Operator/1 -> y/1
  T/1 -> MinMax/1, Relational Operator/2
  MinMax/1 -> Add/2

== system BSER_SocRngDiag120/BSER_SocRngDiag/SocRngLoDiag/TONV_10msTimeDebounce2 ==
  note: Turn On Delay Time Deboune
  u : Inport
  T : Inport  Port=2
  Add : Sum
  Constant1 : Constant  Value=0  OutDataTypeStr=single
  Constant2 : Constant  OutDataTypeStr=uint8
  Constant3 : Constant  Value=0  OutDataTypeStr=uint8
  Constant4 : Constant  Value=0.01  OutDataTypeStr=single
  Delay : Delay  DelayLength=1  InitialCondition=0
  MinMax : MinMax  Inputs=2
  Product : Product  OutMin=[0]  OutMax=[65535]  OutDataTypeStr=single
  Relational Operator : RelationalOperator  Operator=>  OutDataTypeStr=boolean  RndMeth=Simplest
  Switch : Switch  Criteria=u2 ~= 0
  Switch1 : Switch  Criteria=u2 ~= 0
  y : Outport
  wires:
  MinMax/1 -> Add/2
  T/1 -> Relational Operator/2, MinMax/1
  Relational Operator/1 -> y/1
  Delay/1 -> MinMax/2
  Switch/1 -> Add/1
  Product/1 -> Delay/1, Relational Operator/1
  Add/1 -> Product/2
  Constant1/1 -> Switch/3
  Constant4/1 -> Switch/1
  u/1 -> Switch/2, Switch1/2
  Constant2/1 -> Switch1/1
  Constant3/1 -> Switch1/3
  Switch1/1 -> Product/1

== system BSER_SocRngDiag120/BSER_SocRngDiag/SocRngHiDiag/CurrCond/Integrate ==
  In : Inport
  Add : Sum
  Delay : Delay  DelayLength=1  InitialCondition=0
  Gain : Gain  Gain=0.01
  Saturation : Saturate  UpperLimit=0  LowerLimit=-10000
  Out : Outport
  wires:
  Saturation/1 -> Delay/1, Out/1
  In/1 -> Gain/1
  Delay/1 -> Add/1
  Add/1 -> Saturation/1
  Gain/1 -> Add/2

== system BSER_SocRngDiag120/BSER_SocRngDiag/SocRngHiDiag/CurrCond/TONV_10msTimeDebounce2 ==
  note: Turn On Delay Time Deboune
  u : Inport
  T : Inport  Port=2
  Add : Sum
  Constant1 : Constant  Value=0  OutDataTypeStr=single
  Constant2 : Constant  OutDataTypeStr=uint8
  Constant3 : Constant  Value=0  OutDataTypeStr=uint8
  Constant4 : Constant  Value=0.01  OutDataTypeStr=single
  Delay : Delay  DelayLength=1  InitialCondition=0
  MinMax : MinMax  Inputs=2
  Product : Product  OutMin=[0]  OutMax=[65535]  OutDataTypeStr=single
  Relational Operator : RelationalOperator  Operator=>  OutDataTypeStr=boolean  RndMeth=Simplest
  Switch : Switch  Criteria=u2 ~= 0
  Switch1 : Switch  Criteria=u2 ~= 0
  y : Outport
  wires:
  MinMax/1 -> Add/2
  T/1 -> Relational Operator/2, MinMax/1
  Relational Operator/1 -> y/1
  Delay/1 -> MinMax/2
  Switch/1 -> Add/1
  Product/1 -> Delay/1, Relational Operator/1
  Add/1 -> Product/2
  Constant1/1 -> Switch/3
  Constant4/1 -> Switch/1
  u/1 -> Switch/2, Switch1/2
  Constant2/1 -> Switch1/1
  Constant3/1 -> Switch1/3
  Switch1/1 -> Product/1

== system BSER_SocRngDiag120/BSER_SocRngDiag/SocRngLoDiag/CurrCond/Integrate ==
  In : Inport
  Add : Sum
  Delay : Delay  DelayLength=1  InitialCondition=0
  Gain : Gain  Gain=0.01
  Saturation : Saturate  UpperLimit=10000  LowerLimit=0
  Out : Outport
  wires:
  Saturation/1 -> Delay/1, Out/1
  In/1 -> Gain/1
  Delay/1 -> Add/1
  Add/1 -> Saturation/1
  Gain/1 -> Add/2

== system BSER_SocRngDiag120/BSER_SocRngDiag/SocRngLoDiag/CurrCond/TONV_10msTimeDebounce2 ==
  note: Turn On Delay Time Deboune
  u : Inport
  T : Inport  Port=2
  Add : Sum
  Constant1 : Constant  Value=0  OutDataTypeStr=single
  Constant2 : Constant  OutDataTypeStr=uint8
  Constant3 : Constant  Value=0  OutDataTypeStr=uint8
  Constant4 : Constant  Value=0.01  OutDataTypeStr=single
  Delay : Delay  DelayLength=1  InitialCondition=0
  MinMax : MinMax  Inputs=2
  Product : Product  OutMin=[0]  OutMax=[65535]  OutDataTypeStr=single
  Relational Operator : RelationalOperator  Operator=>  OutDataTypeStr=boolean  RndMeth=Simplest
  Switch : Switch  Criteria=u2 ~= 0
  Switch1 : Switch  Criteria=u2 ~= 0
  y : Outport
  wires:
  MinMax/1 -> Add/2
  T/1 -> Relational Operator/2, MinMax/1
  Relational Operator/1 -> y/1
  Delay/1 -> MinMax/2
  Switch/1 -> Add/1
  Product/1 -> Delay/1, Relational Operator/1
  Add/1 -> Product/2
  Constant1/1 -> Switch/3
  Constant4/1 -> Switch/1
  u/1 -> Switch/2, Switch1/2
  Constant2/1 -> Switch1/1
  Constant3/1 -> Switch1/3
  Switch1/1 -> Product/1
